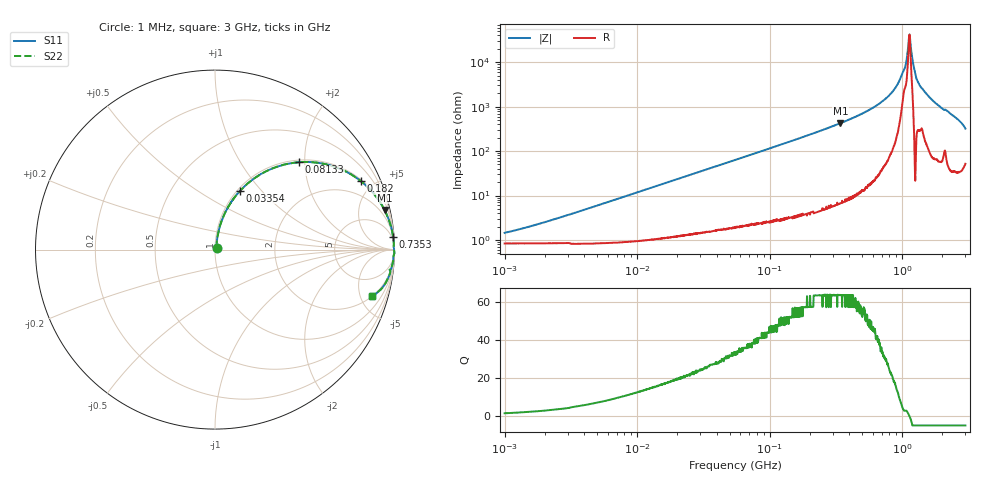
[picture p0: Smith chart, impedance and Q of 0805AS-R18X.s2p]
!s-Parameter Generated by FASTRON Sdn. Bhd.
!FASTRON P/N : 0805AS-R18X
!Keysight Technologies: E4991B_MY54100416_A.01.15
!Date: Mon Jun 15 12:52:43 2026
!Version  :Rev01  Mon Jun 15 12:52:43 2026
!Data & Calibration Information:
!Freq  S11  S21  S12  S22
!PortZ  Port1:50+j0  Port2:50+j0
!When reading reference impedance value at option line is always used.
! Remarks : This data is being provided solely for informational purposes.
# Hz S dB R 50
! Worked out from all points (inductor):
!   1601 points, 1 MHz to 3 GHz, reference 50 ohm
!   read as one part in series: L = 188 nH near 2.14 MHz
!   highest Q = 63.7 at 341.9 MHz (marker M1), where L = 197 nH
!   self-resonance near 1.131 GHz
!   S11 on the Smith chart (normalised r, x): 1 MHz: 1.02, +0.02; 33.54 MHz: 1.03, +0.78; 81.33 MHz: 1.05, +1.87; 182 MHz: 1.07, +4.23; 735.3 MHz: 2, +29; 3 GHz: 2.04, -6.34
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1000000  -36.90 54.1  -0.07 -0.7  -0.07 -0.7  -36.90 54.1
3804036  -26.90 77.1  -0.08 -2.5  -0.08 -2.5  -26.90 77.1
1.447069e7  -15.60 76.9  -0.21 -9.5  -0.21 -9.5  -15.60 76.9
3.354185e7  -8.94 66.8  -0.72 -20.9  -0.72 -20.9  -8.94 66.8
5.504702e7  -5.55 56.4  -1.58 -31.9  -1.58 -31.9  -5.55 56.4
8.132864e7  -3.42 46.2  -2.83 -42.4  -2.83 -42.4  -3.42 46.2
1.820241e8  -0.93 25.1  -7.46 -63.9  -7.46 -63.9  -0.93 25.1
2.083556e8  -0.72 22.1  -8.48 -66.9  -8.48 -66.9  -0.72 22.1
3.419417e8  -0.26 13.2  -12.80 -75.9  -12.80 -75.9  -0.26 13.2
7.352784e8  -0.04 4.0  -23.20 -84.2  -23.20 -84.2  -0.04 4.0
7.925923e8  -0.03 3.2  -24.90 -84.5  -24.90 -84.5  -0.03 3.2
9.072485e8  -0.03 1.9  -29.30 -84.0  -29.30 -84.0  -0.03 1.9
1.01283e9  -0.04 0.9  -35.60 -74.3  -35.60 -74.3  -0.04 0.9
1.059487e9  -0.04 0.6  -38.40 -69.4  -38.40 -69.4  -0.04 0.6
1.108292e9  -0.02 0.2  -46.60 -55.4  -46.60 -55.4  -0.02 0.2
1.136371e9  -0.02 -0.0  -52.50 5.7  -52.50 5.7  -0.02 -0.0
1.165162e9  -0.02 -0.2  -46.40 64.8  -46.40 64.8  -0.02 -0.2
1.218836e9  -0.01 -0.7  -38.40 86.0  -38.40 86.0  -0.01 -0.7
1.268618e9  -0.00 -1.2  -33.50 87.9  -33.50 87.9  -0.00 -1.2
1.388188e9  -0.04 -2.1  -28.70 81.5  -28.70 81.5  -0.04 -2.1
1.747494e9  -0.06 -4.5  -22.20 82.5  -22.20 82.5  -0.06 -4.5
3e9  -0.78 -16.3  -10.90 64.4  -10.90 64.4  -0.78 -16.3
